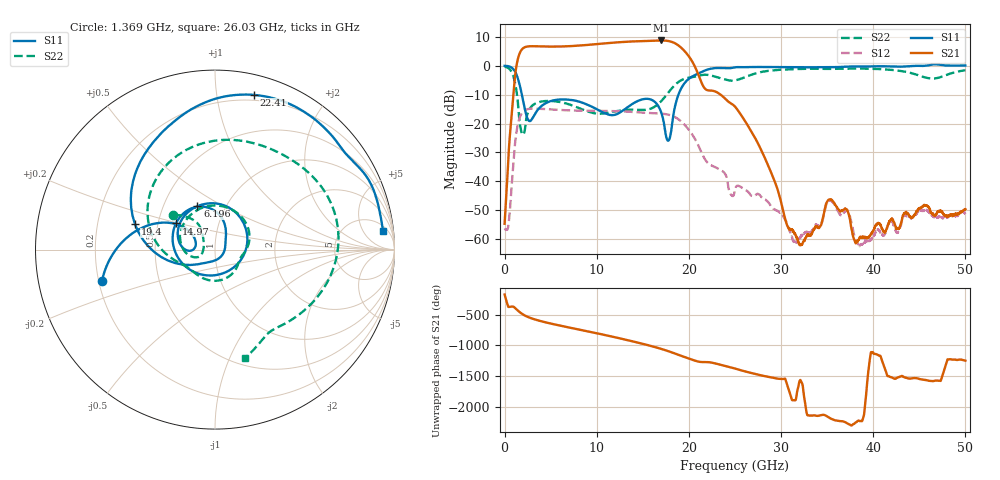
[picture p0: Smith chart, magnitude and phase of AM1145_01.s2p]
!Agilent Technologies,E8364B,MY43040894,A.07.50.67
!Agilent E8364B: A.07.50.67
!Date: Monday, November 15, 2021 11:32:29
!Correction: S11(Full 2 Port(1,2))
!S21(Full 2 Port(1,2))
!S12(Full 2 Port(1,2))
!S22(Full 2 Port(1,2))
!S2P File: Measurements: S11, S21, S12, S22:
# Hz S  dB  R 50
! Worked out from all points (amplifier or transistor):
!   6401 points, 10 MHz to 50 GHz, reference 50 ohm
!   highest |S21| = 8.7 dB at 16.96 GHz (marker M1)
!   |S21| within 3 dB of that: 1.914 GHz to 19.33 GHz (17.42 GHz wide, 164 % of centre)
!   unconditionally stable (mu >= 1): start of sweep to 45.77 GHz
!   at 8.336 GHz: K = 1.41, MAG = 7.5 dB, |S12| = -15.6 dB
!   at 25 GHz: K = 30.03, MAG = -3.4 dB, |S12| = -42.9 dB
!   at 50 GHz: K = -264.75, MSG = 0.9 dB, |S12| = -51.3 dB
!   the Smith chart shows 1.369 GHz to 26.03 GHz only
!   S11 on the Smith chart (normalised r, x): 1.369 GHz: 0.21, -0.13; 6.196 GHz: 0.74, +0.38; 14.97 GHz: 0.62, +0.19; 19.4 GHz: 0.37, +0.13; 22.41 GHz: 0.15, +1.27; 26.03 GHz: 8, +14
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1e7  -0.04 -12.4  -54.68 -169.4  -56.24 -25.9  -0.29 -16.6
1.369103e9  -3.68 -164.4  1.19 -60.2  -21.58 153.1  -10.41 140.2
1.884625e9  -10.04 151.4  5.62 -122.5  -16.41 85.0  -23.38 157.1
2.767261e9  -19.16 170.2  6.72 171.1  -14.91 13.6  -14.73 175.8
4.298205e9  -13.30 162.2  6.64 102.8  -14.99 -57.1  -12.26 105.7
6.196262e9  -11.67 112.2  6.65 38.4  -15.35 -120.1  -12.68 47.4
8.34427e9  -12.69 56.2  7.01 -28.6  -15.57 177.2  -15.00 2.1
1.053914e10  -15.93 -15.0  7.62 -98.1  -15.64 114.1  -16.58 -24.4
1.258561e10  -16.07 -117.3  8.15 -166.7  -15.78 53.1  -15.48 -62.0
1.496795e10  -11.63 146.2  8.50 107.2  -16.23 -21.8  -15.30 -126.9
1.667854e10  -13.95 84.6  8.71 38.3  -16.52 -81.5  -13.27 -161.2
1.695973e10  -15.81 72.4  8.73 25.8  -16.58 -92.4  -12.41 -167.1
1.842819e10  -15.11 -151.1  7.87 -48.4  -17.67 -157.8  -6.87 145.4
1.940456e10  -6.60 162.4  5.49 -102.1  -20.01 153.9  -4.68 103.6
2.084177e10  -2.97 115.6  -1.64 -176.2  -26.38 85.6  -3.66 50.2
2.241177e10  -1.02 76.0  -8.62 161.3  -34.42 52.9  -3.40 -4.8
2.5005e10  -0.56 25.7  -14.15 63.6  -42.88 5.5  -5.10 -59.2
2.602823e10  -0.52 6.0  -18.81 19.3  -42.79 -52.6  -4.04 -74.7
3.333927e10  -0.55 -110.5  -58.08 14.4  -57.26 47.2  -1.06 160.8
4.167354e10  -0.23 158.2  -54.50 -61.7  -54.63 -54.0  -1.37 66.6
4.661005e10  0.49 126.8  -51.91 -139.1  -52.28 -44.0  -4.42 -86.8
5e10  0.07 104.8  -49.58 -168.0  -51.35 -164.8  -1.60 151.7
